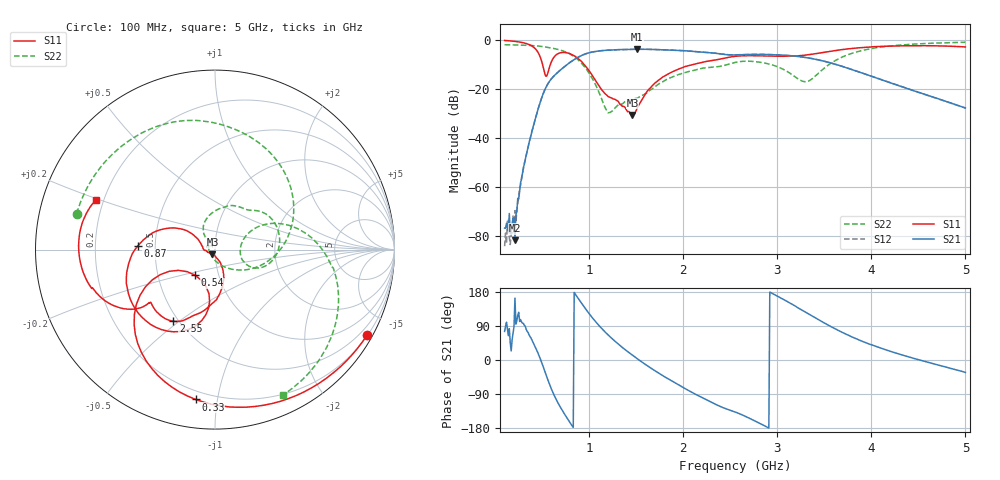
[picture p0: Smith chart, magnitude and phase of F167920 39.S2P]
!  2-Port S-parameters saved by WinCal
! VAR MeasName=S-Parameters (CALIBRATED_DATA) read from VNA (N5242A)
! VAR MeasDate=2016-11-22 9:57:20
! VAR NAME=F167920 39
! VAR FILENAME=F167920 39.S2P
! VAR DATE=2016-11-22 9:57:20
! VAR PHYS_PORTS=1,2
# Hz S DB R 50
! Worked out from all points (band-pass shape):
!   491 points, 100 MHz to 5 GHz, reference 50 ohm
!   highest |S21| = -3.82 dB at 1.51 GHz (marker M1); lowest = -81.6 dB at 210 MHz (marker M2)
!   |S21| within 3 dB of the highest: 894.5 MHz to 3.228 GHz (2.333 GHz wide, 113 % of centre)
!   lowest |S11| = -30.5 dB at 1.46 GHz (marker M3), VSWR 1.06, Z = 48.5 - j2.54 ohm
!   |S11| at or under -10 dB: 503.3 MHz to 586.8 MHz (83.43 MHz wide, 15.3 % of centre); 945.4 MHz to 2.108 GHz (1.163 GHz wide, 76.2 % of centre)
!   |S22| runs from -29.7 to -1.0 dB; largest |S21 - S12| = 0.0022
!   S11 on the Smith chart (normalised r, x): 100 MHz: 0.22, -3.82; 330 MHz: 0.15, -0.87; 540 MHz: 0.77, -0.23; 870 MHz: 0.40, +0.02; 2.55 GHz: 0.47, -0.48; 5 GHz: 0.17, +0.20
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1e8  -0.25 -29.3  -76.62 75.4  -83.98 1.5  -1.98 165.5
1.8e8  -0.50 -52.2  -74.74 53.8  -78.83 75.9  -2.04 153.8
2.1e8  -0.62 -60.9  -81.60 163.5  -69.49 133.1  -2.06 149.3
3.3e8  -1.49 -97.4  -46.95 80.6  -47.01 82.6  -2.21 130.7
4.4e8  -4.24 -137.3  -30.31 26.9  -30.26 27.0  -2.46 111.8
5.4e8  -14.86 -127.9  -19.31 -38.7  -19.31 -38.6  -2.94 92.8
6.7e8  -5.58 -120.4  -13.06 -114.3  -13.05 -114.3  -3.93 65.3
7.7e8  -5.34 -153.1  -9.91 -155.5  -9.90 -155.6  -5.25 39.5
8.7e8  -7.29 177.5  -7.33 167.0  -7.32 167.0  -7.73 9.6
9.2e8  -8.88 164.9  -6.31 149.3  -6.31 149.2  -9.62 -6.5
1.06e9  -16.14 145.6  -4.76 103.4  -4.76 103.4  -17.71 -53.8
1.2e9  -23.04 167.3  -4.19 66.2  -4.19 66.2  -29.69 -146.0
1.46e9  -30.54 -118.3  -3.86 12.6  -3.86 12.7  -24.25 122.0
1.51e9  -27.72 -83.3  -3.82 3.4  -3.82 3.5  -23.76 122.9
1.74e9  -16.30 -71.6  -3.99 -34.9  -3.98 -34.9  -17.98 121.4
2.08e9  -10.27 -94.0  -4.61 -83.8  -4.60 -83.8  -12.70 82.4
2.55e9  -6.71 -120.2  -6.13 -137.0  -6.11 -137.1  -9.19 34.6
2.96e9  -6.64 -139.2  -6.05 174.0  -6.04 173.8  -10.37 -16.4
3.37e9  -5.85 -141.5  -7.64 116.1  -7.60 116.0  -15.86 17.2
3.7e9  -3.90 -150.3  -10.92 71.8  -10.90 71.5  -6.83 16.1
4.19e9  -2.55 -170.6  -17.32 23.9  -17.32 23.5  -2.54 -22.8
5e9  -2.89 157.1  -27.73 -32.7  -27.77 -33.1  -0.97 -65.1
